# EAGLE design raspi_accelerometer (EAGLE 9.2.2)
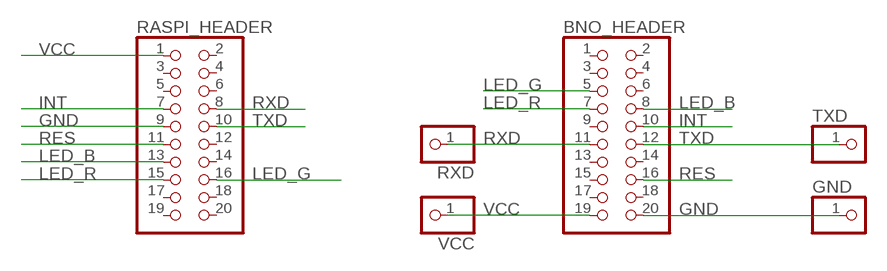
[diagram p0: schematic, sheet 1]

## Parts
BNO_HEADER  PINHD-2X10/90  [2X10/90]
GND  PINHD-1X1  [1X01]
RASPI_HEADER  PINHD-2X10  [2X10]
RXD  PINHD-1X1  [1X01]
TXD  PINHD-1X1  [1X01]
VCC  PINHD-1X1  [1X01]

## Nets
GND: BNO_HEADER.20 GND.1 RASPI_HEADER.9
INT: BNO_HEADER.10 RASPI_HEADER.7
LED_B: BNO_HEADER.8 RASPI_HEADER.13
LED_G: BNO_HEADER.5 RASPI_HEADER.16
LED_R: BNO_HEADER.7 RASPI_HEADER.15
RES: BNO_HEADER.16 RASPI_HEADER.11
RXD: BNO_HEADER.11 RASPI_HEADER.8 RXD.1
TXD: BNO_HEADER.12 RASPI_HEADER.10 TXD.1
VCC: BNO_HEADER.19 RASPI_HEADER.1 VCC.1
Unconnected: BNO_HEADER.1 BNO_HEADER.2 BNO_HEADER.3 BNO_HEADER.4 BNO_HEADER.6 BNO_HEADER.9 BNO_HEADER.13 BNO_HEADER.14 BNO_HEADER.15 BNO_HEADER.17 BNO_HEADER.18 RASPI_HEADER.2 RASPI_HEADER.3 RASPI_HEADER.4 RASPI_HEADER.5 RASPI_HEADER.6 RASPI_HEADER.12 RASPI_HEADER.14 RASPI_HEADER.17 RASPI_HEADER.18 RASPI_HEADER.19 RASPI_HEADER.20

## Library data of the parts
BNO_HEADER RASPI_HEADER = pinhead:PINHD-2X10: PIN HEADER
GND RXD TXD VCC = pinhead:PINHD-1X1: PIN HEADER

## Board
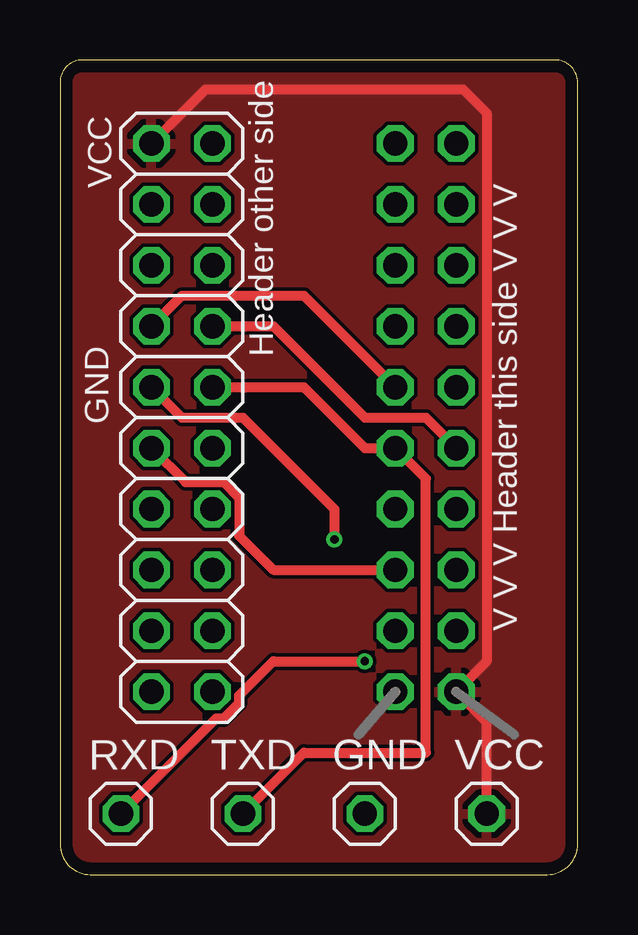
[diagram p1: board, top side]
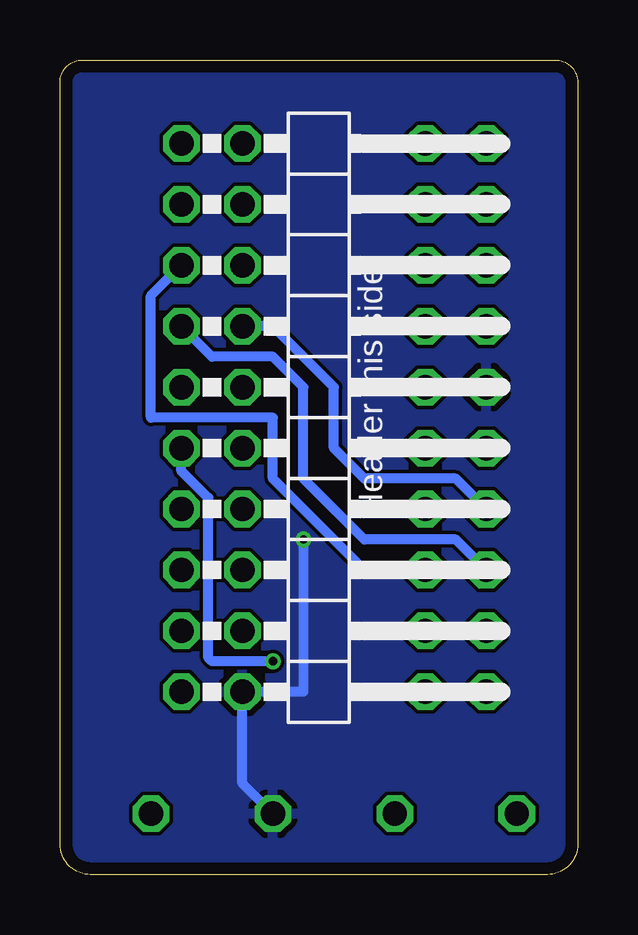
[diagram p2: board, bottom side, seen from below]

Size 21.57 x 33.96 mm. Coordinates in mm from the lower left corner, seen from the top.
Outline: 1.27,0 20.3,0 arc90 21.57,1.27 21.57,33.02 arc90 20.63,33.96 0.94,33.96 arc90 0,33.02 0,1.27 arc90 1.27,0
Copper layers (1*16): Top 0.035mm / dielectric 1.6mm / Bottom 0.035mm
Design rules "Elecrow_2-layer_PCB_eagle_rule": minimum track width 6mil, minimum drill 12mil, track to track 6mil, track to pad 6mil, pad to pad 6mil, via to via 8mil, smd to smd 0mil, copper to edge 20mil, drill to drill 10mil, minimum pad ring 6mil, minimum via ring 6mil, stop-mask expansion 0mil, vias tented up to drill 100mil, thermal gap 10mil

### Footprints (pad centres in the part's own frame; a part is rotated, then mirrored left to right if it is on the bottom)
2X10/90 = drill 1.016 octagon: 1 -11.43,-6.35; 2 -11.43,-3.81; 3 -8.89,-6.35; 4 -8.89,-3.81; 5 -6.35,-6.35; 6 -6.35,-3.81; 7 -3.81,-6.35; 8 -3.81,-3.81; 9 -1.27,-6.35; 10 -1.27,-3.81; 11 1.27,-6.35; 12 1.27,-3.81; 13 3.81,-6.35; 14 3.81,-3.81; 15 6.35,-6.35; 16 6.35,-3.81; 17 8.89,-6.35; 18 8.89,-3.81; 19 11.43,-6.35; 20 11.43,-3.81
1X01 = drill 1.016 octagon: 1 0,0
2X10 = drill 1.016 octagon: 1 -11.43,-1.27; 2 -11.43,1.27; 3 -8.89,-1.27; 4 -8.89,1.27; 5 -6.35,-1.27; 6 -6.35,1.27; 7 -3.81,-1.27; 8 -3.81,1.27; 9 -1.27,-1.27; 10 -1.27,1.27; 11 1.27,-1.27; 12 1.27,1.27; 13 3.81,-1.27; 14 3.81,1.27; 15 6.35,-1.27; 16 6.35,1.27; 17 8.89,-1.27; 18 8.89,1.27; 19 11.43,-1.27; 20 11.43,1.27

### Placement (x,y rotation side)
BNO_HEADER  10.16,19.05 270 bottom
GND  12.7,2.54 0 top
RASPI_HEADER  5.08,19.05 270 top
RXD  2.54,2.54 0 top
TXD  7.62,2.54 0 top
VCC  17.78,2.54 0 top

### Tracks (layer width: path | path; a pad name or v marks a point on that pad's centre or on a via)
GND  (via drill 0.35)
  Top 0.406: RASPI_HEADER.9 5.08,19.05 7.62,19.05 11.43,15.24 v11.43,13.97
  Bottom 0.406: GND.1 13.97,3.81 BNO_HEADER.20 11.43,7.62 v11.43,13.97
  pour Bottom: 0,34.29 0,0 21.59,0 21.59,34.29
INT
  Top 0.406: RASPI_HEADER.7 5.08,24.13 10.16,24.13 BNO_HEADER.10
LED_B
  Bottom 0.406: RASPI_HEADER.13 5.08,16.51 8.89,16.51 10.16,17.78 10.16,20.32 12.7,22.86 BNO_HEADER.8
LED_G
  Bottom 0.406: RASPI_HEADER.16 8.89,12.7 12.7,16.51 12.7,19.05 17.78,19.05 17.78,24.13 BNO_HEADER.5
LED_R
  Bottom 0.406: RASPI_HEADER.15 5.08,13.97 8.89,13.97 11.43,16.51 11.43,20.32 12.7,21.59 15.24,21.59 BNO_HEADER.7
RES
  Top 0.406: BNO_HEADER.16 8.89,12.7 7.47,14.12 7.47,15.7 6.81,16.36 5.23,16.36 RASPI_HEADER.11
RXD  (via drill 0.35)
  Top 0.406: v12.7,8.89 8.89,8.89 7.47,7.47 7.47,7.16 6.81,6.5 6.5,6.5 RXD.1 | RASPI_HEADER.8 8.89,22.86 12.7,19.05 15.24,19.05 BNO_HEADER.11
  Bottom 0.406: v12.7,8.89 15.24,8.89 15.39,9.04 15.39,15.7 16.51,16.82 BNO_HEADER.11
TXD
  Top 0.406: TXD.1 10.16,5.08 15.24,5.08 15.24,16.51 BNO_HEADER.12 12.7,17.78 10.16,20.32 RASPI_HEADER.10
VCC
  Top 0.406: RASPI_HEADER.1 6.07,32.74 16.79,32.74 17.78,31.75 17.78,8.89 BNO_HEADER.19 17.78,6.35 VCC.1
  pour Top: 0,34.29 0,0 21.59,0 21.59,34.29

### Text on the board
tPlace: VCC | GND | V V V Header this side V V V
tNames: Header other side
bNames: Header this side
